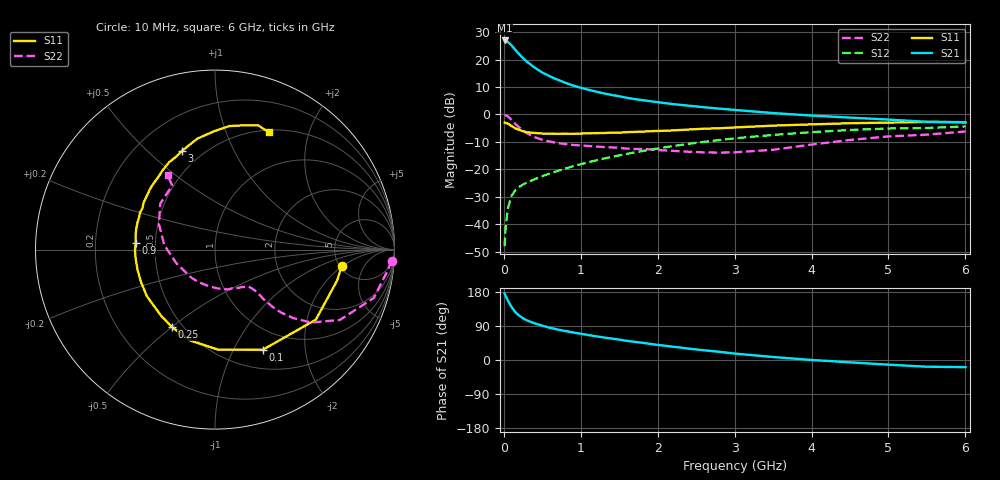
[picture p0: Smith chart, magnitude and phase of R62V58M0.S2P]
! SIEMENS Small Signal Semiconductors
! BFR193
! Si NPN RF Bipolar Junction Transistor in SOT23
! VCE = 2.5 V  IC = 8 mA
! Common Emitter S-Parameters:  May  1996
# GHz  S  MA  R  50
!  f  S11  S21  S12  S22
! GHz  MAG  ANG  MAG  ANG  MAG  ANG  MAG  ANG
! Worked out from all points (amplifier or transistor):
!   36 points, 10 MHz to 6 GHz, reference 50 ohm
!   highest |S21| = 26.9 dB at 10 MHz (marker M1)
!   |S21| within 3 dB of that: start of sweep to 136.9 MHz
!   unconditionally stable (mu >= 1): 778.6 MHz to 1.967 GHz
!   at 250 MHz: K = 0.57, MSG = 23.0 dB, |S12| = -25.5 dB
!   at 1.4 GHz: K = 1.04, MAG = 10.0 dB, |S12| = -15.5 dB
!   at 6 GHz: K = 0.95, MSG = 0.8 dB, |S12| = -4.4 dB
!   lowest NFmin = 1.25 dB at 450 MHz
!   S11 on the Smith chart (normalised r, x): 10 MHz: 5.20, -1.93; 100 MHz: 0.73, -1.31; 250 MHz: 0.44, -0.50; 900 MHz: 0.39, +0.03; 3 GHz: 0.39, +0.64; 6 GHz: 0.53, +1.42
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0.01  0.7119 -7.4  22.26 175.6  0.004 87.9  0.986 -3.6
0.02  0.7019 -14.2  22.24 170.6  0.0076 84.9  0.9683 -7.0
0.05  0.6841 -34.8  21.12 157.7  0.019 74.6  0.9252 -16.9
0.1  0.6183 -64.5  18.09 139.9  0.033 63.3  0.7985 -29.4
0.15  0.5578 -88.2  15 126.2  0.042 56.9  0.6721 -37.2
0.2  0.5253 -104.9  12.51 117.1  0.0481 54.2  0.5796 -41.2
0.25  0.4942 -118.9  10.59 109.9  0.0531 52.7  0.5082 -43.6
0.3  0.4745 -129.6  9.155 104.6  0.0578 52.8  0.455 -44.8
0.4  0.4598 -145.7  7.146 96.8  0.0662 53.9  0.3863 -45.6
0.5  0.4502 -156.4  5.79 90.5  0.0752 55.3  0.3464 -45.4
0.6  0.4462 -165.5  4.929 85.1  0.0843 57.2  0.3202 -45.7
0.7  0.4447 -173.1  4.282 80.4  0.0935 58.6  0.3022 -46.3
0.9  0.4436 175.4  3.365 72.6  0.1141 60.0  0.2783 -47.8
1.1  0.4535 165.7  2.817 65.8  0.1351 61.0  0.2668 -51.3
1.3  0.4595 157.2  2.417 59.4  0.1575 60.7  0.2552 -55.1
1.6  0.4764 146.5  2.012 50.5  0.1919 59.7  0.2392 -63.5
2.2  0.5121 128.4  1.542 35.1  0.2659 54.6  0.2177 -85.1
3  0.5797 108.6  1.21 17.0  0.3678 44.3  0.2044 -128.9
3.5  0.6263 99.0  1.06 7.9  0.4237 36.6  0.2275 -159.9
4.5  0.6929 83.4  0.877 -6.2  0.5216 21.2  0.3433 155.6
5.5  0.7327 70.8  0.734 -17.7  0.5672 5.2  0.429 123.8
6  0.7192 65.4  0.725 -18.8  0.6052 0.6  0.4899 122.5
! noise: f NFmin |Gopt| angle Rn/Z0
0.45  1.25  0.23  133  0.12
0.9  1.3  0.35  156  0.11
1.8  2  0.55  -155  0.13
